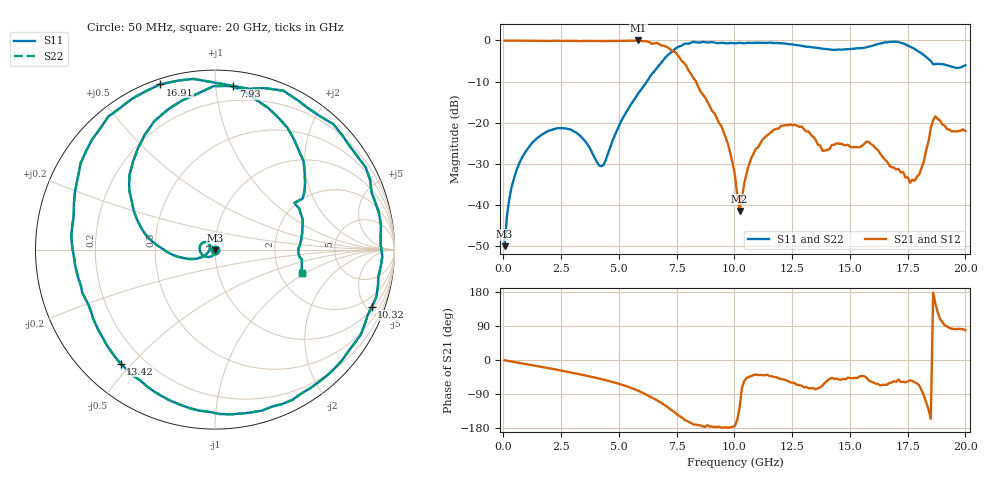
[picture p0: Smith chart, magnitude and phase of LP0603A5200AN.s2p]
!	AVX THIN FILM OPERATION
!	0603 SIZE LOW PASS FILTER P/N LP0603N5200ANTR
!	Created August 2007
!	Network Analyzer HP8720E S.07.64: Feb23, 2000 Serial No.US39172382
#	mhz	S	db	R	50
!	S11	S11	S21	S21	S12	S12	S22	S22
!	dB	Phase	dB	Phase	dB	Phase	dB	Phase
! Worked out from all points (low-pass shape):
!   201 points, 50 MHz to 20 GHz, reference 50 ohm
!   highest |S21| = 0.01 dB at 5.835 GHz (marker M1); lowest = -41.4 dB at 10.22 GHz (marker M2)
!   |S21| within 3 dB of the highest: start of sweep to 7.464 GHz
!   lowest |S11| = -50.0 dB at 50 MHz (marker M3), VSWR 1.01, Z = 50.3 - j0.176 ohm
!   |S11| at or under -10 dB: start of sweep to 6.207 GHz
!   |S22| runs from -50.0 to -0.3 dB; largest |S21 - S12| = 0
!   S11 on the Smith chart (normalised r, x): 50 MHz: 1.01, -0.00; 7.93 GHz: 0.10, +1.11; 10.32 GHz: 1.15, -5.39; 13.42 GHz: 0.12, -0.47; 16.91 GHz: 0.02, +0.72; 20 GHz: 2.65, -0.90
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50  -49.98 -33.5  -0.04 -0.7  -0.04 -0.7  -49.98 -33.5
349.25  -35.70 -88.3  -0.05 -3.8  -0.05 -3.8  -35.70 -88.3
1047.5  -26.32 -125.0  -0.05 -11.4  -0.05 -11.4  -26.32 -125.0
3441.5  -23.85 139.4  -0.11 -39.6  -0.11 -39.6  -23.85 139.4
4339.25  -30.21 -175.8  -0.13 -52.1  -0.13 -52.1  -30.21 -175.8
5835.5  -12.85 -171.5  0.01 -81.1  0.01 -81.1  -12.85 -171.5
6733.25  -6.05 154.9  -0.84 -109.8  -0.84 -109.8  -6.05 154.9
7331.75  -2.51 121.6  -2.67 -134.7  -2.67 -134.7  -2.51 121.6
7930.25  -0.75 83.6  -6.35 -160.5  -6.35 -160.5  -0.75 83.6
9027.5  -0.39 28.6  -17.09 -175.7  -17.09 -175.7  -0.39 28.6
10025  -0.70 -9.4  -32.76 -173.1  -32.76 -173.1  -0.70 -9.4
10224.5  -0.56 -16.4  -41.42 -124.9  -41.42 -124.9  -0.56 -16.4
10324.25  -0.64 -20.1  -38.24 -73.9  -38.24 -73.9  -0.64 -20.1
11321.75  -0.56 -55.4  -23.51 -40.2  -23.51 -40.2  -0.56 -55.4
12219.5  -0.76 -88.5  -20.58 -53.0  -20.58 -53.0  -0.76 -88.5
13416.5  -1.68 -129.6  -23.45 -74.1  -23.45 -74.1  -1.68 -129.6
15311.75  -1.88 174.2  -25.94 -47.5  -25.94 -47.5  -1.88 174.2
16708.25  -0.36 118.6  -30.37 -60.3  -30.37 -60.3  -0.36 118.6
16907.75  -0.27 108.5  -30.89 -55.9  -30.89 -55.9  -0.27 108.5
18104.75  -3.13 44.9  -30.84 -80.1  -30.84 -80.1  -3.13 44.9
18703.25  -5.75 28.3  -18.39 148.1  -18.39 148.1  -5.75 28.3
20000  -6.03 -14.8  -22.04 78.8  -22.04 78.8  -6.03 -14.8
